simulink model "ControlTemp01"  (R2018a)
settings: Solver=VariableStepAuto  StartTime=0.0  StopTime=15  RelTol=1e-3
undefined symbols (not defined in the file): ControlTemp01, sdiscope

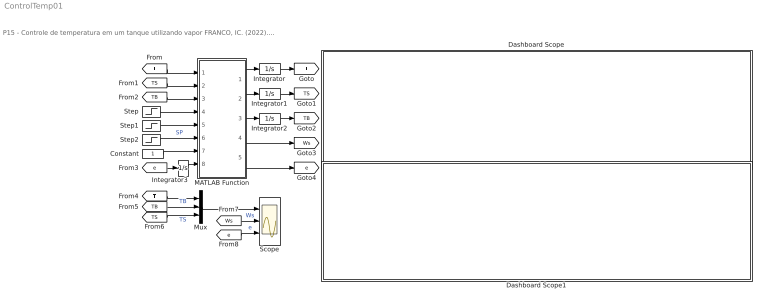
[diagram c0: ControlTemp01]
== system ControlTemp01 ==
  note: P15 - Controle de temperatura em um tanque utilizando vapor FRANCO, IC. (2022). Modelagem e Simulação: Problemas Típicos da Engenharia Química para Simulação e Análise. NOTAS DE AULA INOVADORAS. The Journal of Engineering and Exact Sciences. Material Complementar.
  Constant : Constant
  Dashboard Scope : Subsystem  DialogController=hmiCreateDDGDialog  IsWebBlock=on  mask(MWDashboardBlock){webBlockId=96459436-56d7-49e0-bfcc-bfb577f7875d, webBlockType=sdiscope, ShowInitialText=on, HMISrcModelName=ControlTemp01}
      mask prompts: webBlockId "WebBlock Id"; webBlockType "WebBlock Type"; HMISrcModelName "Source Model"
      mask help: SimulinkHMI:dialogs:HMIScopeDialogDesc
  Dashboard Scope1 : Subsystem  DialogController=hmiCreateDDGDialog  IsWebBlock=on  mask(MWDashboardBlock){webBlockId=284c8313-1dc5-45bd-9a76-02346d8f5405, webBlockType=sdiscope, ShowInitialText=on, HMISrcModelName=ControlTemp01}
      mask prompts: webBlockId "WebBlock Id"; webBlockType "WebBlock Type"; HMISrcModelName "Source Model"
      mask help: SimulinkHMI:dialogs:HMIScopeDialogDesc
  Integrator : Integrator  InitialCondition=20
  Integrator1 : Integrator  InitialCondition=20
  Integrator2 : Integrator  InitialCondition=20
  Integrator3 : Integrator
  MATLAB Function : MATLAB Function  TreatAsAtomicUnit=on
  Mux : Mux  Inputs=3
  Scope : Scope  NumInputPorts=3
  Step : Step  Time=0  Before=20  After=20  SampleTime=0
  Step1 : Step  Time=0  Before=250  After=250  SampleTime=0
  Step2 : Step  Time=0  Before=40  After=40  SampleTime=0
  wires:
  [T] -> Mux/1  "T"
  [TB] -> Mux/2  "TB"
  Mux/1 -> Scope/1
  [TS] -> Mux/3  "TS"
  [Ws] -> Scope/2  "Ws"
  [e] -> Scope/3  "e"
  Step1/1 -> MATLAB Function/5(W)
  [T] -> MATLAB Function/1(T)
  Step2/1 -> MATLAB Function/6(Tsp)  "SP"
  MATLAB Function/5(e) -> [e]
  [e] -> Integrator3/1
  MATLAB Function/3(dTB) -> Integrator2/1
  [TS] -> MATLAB Function/2(TS)
  MATLAB Function/4(Ws) -> [Ws]
  Integrator/1 -> [T]
  MATLAB Function/2(dTS) -> Integrator1/1
  Integrator3/1 -> MATLAB Function/8(ie)
  Integrator2/1 -> [TB]
  MATLAB Function/1(dT) -> Integrator/1
  Integrator1/1 -> [TS]
  Step/1 -> MATLAB Function/4(T0)
  [TB] -> MATLAB Function/3(TB)
  Constant/1 -> MATLAB Function/7(KC)

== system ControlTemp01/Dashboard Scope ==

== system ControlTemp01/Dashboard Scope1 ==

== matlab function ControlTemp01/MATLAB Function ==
function [dT,dTS,dTB,Ws,e] = fcn(T,TS,TB,T0,W,Tsp,KC,ie)
%parâmetros
Cp   =   1.0;
m    =  50.0;  
L    = 537.0;
Ws0  =   5.0;
tauB =   0.3;
tauS =   0.1;

%% controlador PI
%parâmetros do controlador
taui =   5.0;
%error
e=Tsp-TS;
%variável manipulada
Ws=Ws0+KC*e+(KC/taui)*ie;

%modelo matemático
dT = (W*Cp*(T0-T)+Ws*L)/(m*Cp);
dTS= (TB-TS)/tauS;
dTB= (T-TB)/tauB;
end
